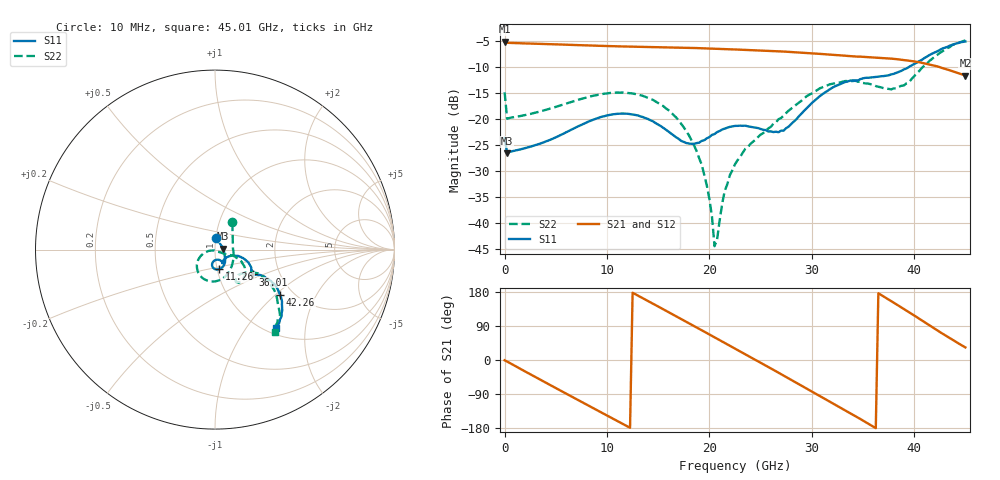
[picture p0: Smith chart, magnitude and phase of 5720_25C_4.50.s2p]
! Device:  ADRF5720
! Description: 0.5dB LSB GaAs MMIC 6-bit Digital Attenuator
! Frequency:  0.000009 -  40 GHz
! Ports:
!	RF1	= Port 1
!	RF2	= Port 2
! Vdd:  3.3 Volt
! Vss:  -3.3 Volt
! Control:  0/3.3 Volt
! State:  4.50 dB attenuation
! Data:  The device was measured using G-S-G Probes on a matrix board.
!  Data was collected using an calibrated 4 port network analyzer.
!  The reference plane for this measurement is at the launchers.
! Note:  Analog Devices supplies this data as a sample of measured data
!  for this product.  Your particular data for this product may vary.
!  Data was taken at 25 degrees C.
!  Analog Devices reserves the right to change this data at anytime.
# GHZ S DB R 45.0
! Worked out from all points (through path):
!   181 points, 10 MHz to 45.01 GHz, reference 45 ohm
!   highest |S21| = -5.22 dB at 10 MHz (marker M1); lowest = -11.7 dB at 45.01 GHz (marker M2)
!   group delay of S21, straight-line fit = 42 ps
!   lowest |S11| = -26.6 dB at 260 MHz (marker M3), VSWR 1.10, Z = 49.4 + j0.476 ohm
!   |S11| at or under -10 dB: start of sweep to 39.54 GHz
!   |S22| runs from -44.4 to -5.0 dB; largest |S21 - S12| = 0.00063
!   S11 on the Smith chart (normalised r, x): 10 MHz: 1.01, +0.13; 11.26 GHz: 1.02, -0.23; 36.01 GHz: 1.45, -0.43; 42.26 GHz: 1.71, -1.09; 45.01 GHz: 1.11, -1.40
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0.01  -23.67 83.7  -5.22 -0.8  -5.22 -0.8  -14.90 57.4
0.26  -26.59 5.9  -5.41 -4.1  -5.41 -4.1  -19.99 1.1
4.26  -24.18 -30.4  -5.66 -63.1  -5.66 -63.1  -18.15 -37.8
7.76  -20.90 -51.8  -5.89 -114.0  -5.88 -114.0  -16.02 -67.2
11.26  -19.01 -78.8  -6.10 -164.5  -6.10 -164.4  -14.97 -98.7
15.26  -21.39 -101.1  -6.25 137.5  -6.25 137.5  -17.24 -137.4
17.51  -24.43 -90.9  -6.36 104.4  -6.36 104.4  -21.63 -157.2
19.26  -24.24 -69.7  -6.46 78.5  -6.45 78.5  -28.78 -168.4
20.01  -23.51 -63.7  -6.51 67.4  -6.51 67.4  -35.41 -161.5
20.51  -22.92 -62.0  -6.54 59.9  -6.54 60.0  -44.44 -126.0
20.76  -22.54 -61.3  -6.56 56.2  -6.56 56.2  -43.18 -82.9
21.51  -21.87 -60.6  -6.62 45.1  -6.62 45.1  -33.82 -34.5
22.76  -21.35 -61.5  -6.71 26.5  -6.71 26.5  -27.95 -25.5
25.01  -21.95 -57.7  -6.89 -7.1  -6.89 -7.1  -23.03 -24.2
27.26  -22.26 -33.3  -7.09 -41.1  -7.09 -41.1  -19.39 -18.3
30.26  -16.55 -15.8  -7.45 -87.0  -7.46 -87.0  -14.78 -28.7
33.51  -12.84 -27.7  -7.93 -136.8  -7.94 -136.8  -12.74 -47.9
36.01  -12.00 -33.5  -8.21 -175.8  -8.22 -175.8  -13.46 -56.8
37.76  -11.48 -31.7  -8.45 155.7  -8.46 155.7  -14.35 -47.3
40.26  -9.23 -29.1  -9.05 113.1  -9.05 113.2  -11.28 -28.9
42.26  -7.05 -35.0  -9.93 78.4  -9.94 78.4  -7.73 -35.2
45.01  -5.15 -51.9  -11.69 33.2  -11.69 33.2  -4.96 -54.0
